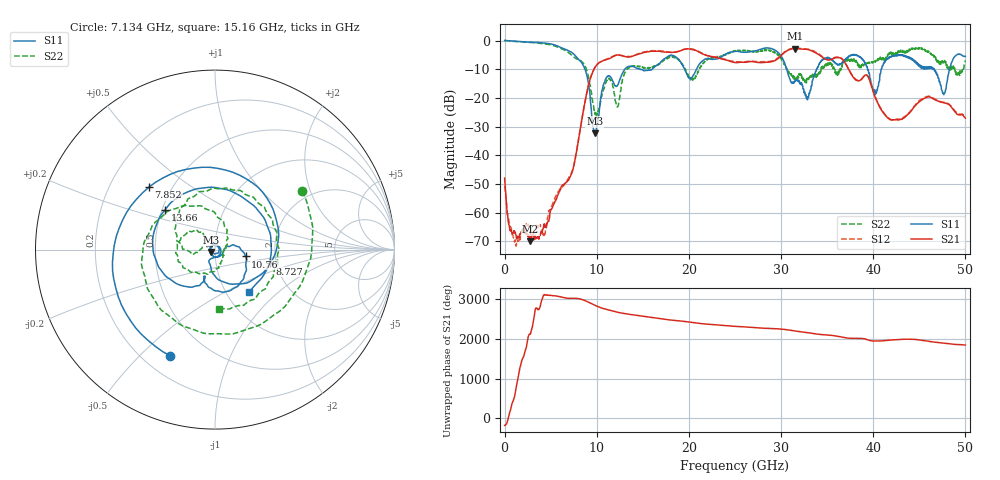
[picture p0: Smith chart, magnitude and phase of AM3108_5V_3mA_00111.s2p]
# Hz S DB R 50.0
!freq dBS11 angS11 dBS21 angS21 dBS12 angS12 dBS22 angS22
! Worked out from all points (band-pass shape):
!   1601 points, 10 MHz to 50 GHz, reference 50 ohm
!   highest |S21| = -2.78 dB at 31.53 GHz (marker M1); lowest = -70.0 dB at 2.791 GHz (marker M2)
!   |S21| within 3 dB of the highest: 11.68 GHz to 22.73 GHz (11.06 GHz wide, 64.3 % of centre); 29.84 GHz to 34.46 GHz (4.625 GHz wide, 14.4 % of centre)
!   lowest |S11| = -32.4 dB at 9.789 GHz (marker M3), VSWR 1.05, Z = 48 - j1.24 ohm
!   |S11| at or under -10 dB: 8.728 GHz to 13.05 GHz (4.325 GHz wide, 39.7 % of centre); 30.63 GHz to 33.85 GHz (3.219 GHz wide, 9.99 % of centre); 46.63 GHz to 48.29 GHz (1.658 GHz wide, 3.49 % of centre)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
!   |S22| runs from -26.6 to 0.0 dB; largest |S21 - S12| = 0.027
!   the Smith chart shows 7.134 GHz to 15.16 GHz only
!   S11 on the Smith chart (normalised r, x): 7.134 GHz: 0.31, -0.62; 7.852 GHz: 0.37, +0.35; 8.727 GHz: 1.85, -0.32; 10.76 GHz: 1.41, -0.11; 13.66 GHz: 0.52, +0.26; 15.16 GHz: 1.27, -0.66
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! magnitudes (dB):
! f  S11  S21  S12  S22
! 10 MHz  0.0  -48.0  -50.7  0.0
! 1.041 GHz  -0.2  -66.7  -69.7  -0.3
! 2.791 GHz  -0.6  -70.0  -67.5  -0.7
! 4.322 GHz  -0.9  -64.0  -67.6  -1.1
! 7.134 GHz  -3.8  -47.5  -46.9  -4.7
! 7.852 GHz  -5.9  -38.0  -37.9  -6.4
! 8.352 GHz  -7.6  -28.2  -28.1  -7.2
! 8.727 GHz  -10.0  -21.4  -21.4  -8.7
! 9.789 GHz  -32.4  -9.5  -9.4  -24.3
! 10.76 GHz  -15.2  -6.9  -6.9  -16.8
! 12.26 GHz  -15.6  -5.0  -5.1  -23.2
! 13.66 GHz  -9.0  -5.7  -5.6  -9.1
! 15.16 GHz  -10.4  -4.1  -4.0  -9.5
! 16.69 GHz  -8.3  -3.7  -3.5  -8.5
! 25 GHz  -3.8  -7.7  -7.3  -3.7
! 31.53 GHz  -14.1  -2.8  -2.6  -13.8
! 33.35 GHz  -15.5  -3.6  -3.3  -12.7
! 38 GHz  -4.8  -13.5  -13.3  -6.5
! 40.22 GHz  -18.8  -19.8  -19.6  -7.6
! 41.69 GHz  -6.0  -27.2  -27.1  -5.2
! 47.66 GHz  -18.9  -21.7  -21.6  -7.7
! 50 GHz  -5.5  -27.0  -26.4  -6.9
